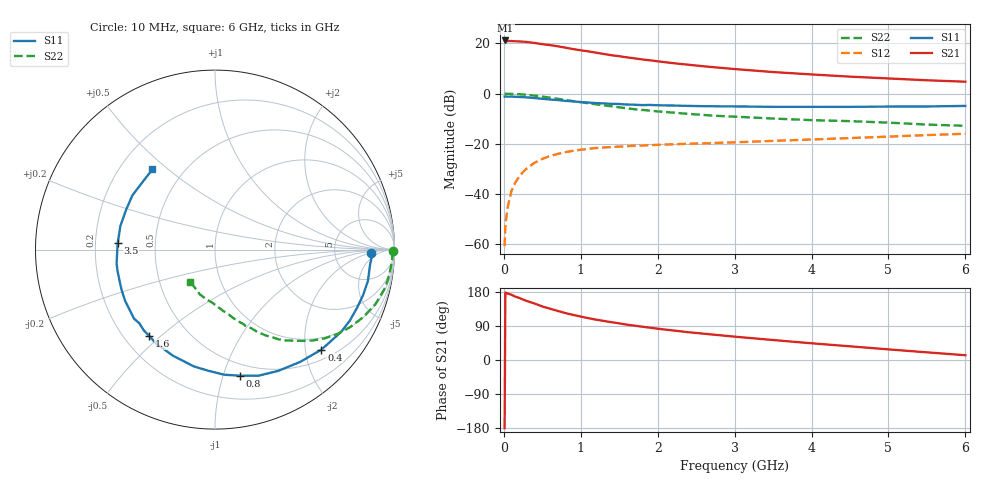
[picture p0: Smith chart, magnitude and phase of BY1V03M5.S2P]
! SIEMENS Small Signal Semiconductors
! BFY420
! Si NPN RF SIEGET Grounded Emitter Transistor in MICRO-X
! VCE = 1 V  IC = 3.5 mA
! Common Emitter S-Parameters:  October  1996
# GHz  S  MA  R  50
!  f  S11  S21  S12  S22
! GHz  MAG  ANG  MAG  ANG  MAG  ANG  MAG  ANG
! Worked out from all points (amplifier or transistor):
!   36 points, 10 MHz to 6 GHz, reference 50 ohm
!   highest |S21| = 21.2 dB at 20 MHz (marker M1)
!   |S21| within 3 dB of that: start of sweep to 822.3 MHz
!   unconditionally stable (mu >= 1): 3.395 GHz to end of sweep
!   at 250 MHz: K = 0.09, MSG = 26.0 dB, |S12| = -31.3 dB
!   at 1.4 GHz: K = 0.45, MSG = 18.3 dB, |S12| = -21.4 dB
!   at 6 GHz: K = 1.20, MAG = 7.7 dB, |S12| = -16.0 dB
!   S11 on the Smith chart (normalised r, x): 10 MHz: 14, -2; 400 MHz: 0.71, -2.34; 800 MHz: 0.39, -1.14; 1.6 GHz: 0.30, -0.46; 3.5 GHz: 0.30, +0.03; 6 GHz: 0.34, +0.44
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0.01  0.8711 -1.3  11.42 -179.9  0.0009 86.1  0.9923 -0.6
0.02  0.8749 -2.5  11.48 177.9  0.0024 87.3  0.9896 -1.2
0.05  0.868 -5.6  11.18 175.4  0.0054 88.5  0.9886 -3.1
0.1  0.8697 -11.5  11.16 172.1  0.0115 84.9  0.9838 -6.4
0.15  0.8633 -16.9  11.05 167.0  0.0168 79.9  0.9777 -9.7
0.2  0.8556 -22.1  10.96 163.9  0.022 77.2  0.9707 -12.7
0.25  0.8491 -27.8  10.88 159.5  0.0273 73.6  0.9566 -15.8
0.3  0.8392 -33.1  10.69 155.6  0.0322 71.8  0.9432 -18.9
0.4  0.8138 -43.2  10.23 149.0  0.0417 66.1  0.9076 -24.5
0.5  0.7854 -52.8  9.676 141.3  0.0496 61.3  0.8693 -29.7
0.6  0.7621 -62.4  9.26 135.4  0.0568 56.8  0.8289 -34.5
0.8  0.7159 -78.9  8.248 123.9  0.0677 49.0  0.7448 -42.8
0.9  0.6988 -85.8  7.725 119.0  0.0722 46.1  0.7068 -46.0
1.1  0.6615 -100.3  6.948 110.4  0.0791 40.8  0.64 -52.2
1.3  0.6359 -111.7  6.172 103.1  0.0841 36.5  0.5807 -57.0
1.6  0.6045 -127.3  5.275 93.2  0.0893 32.1  0.5085 -63.3
2.2  0.5767 -150.2  4.044 77.9  0.0973 26.7  0.4169 -72.5
2.8  0.556 -167.2  3.284 65.5  0.1041 24.2  0.357 -79.9
3.5  0.5434 176.3  2.688 52.7  0.1136 22.4  0.3174 -87.6
4.5  0.5427 155.9  2.176 36.1  0.1294 18.6  0.2814 -99.9
5.5  0.5525 136.4  1.842 20.2  0.1484 14.2  0.2405 -117.5
6  0.567 127.9  1.725 12.6  0.1578 11.6  0.227 -128.3
